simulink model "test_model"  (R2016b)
settings: Solver=VariableStepAuto  StartTime=0.0  StopTime=runtime  RelTol=1e-3
InitFcn:
  | clear mex
  | delete test_model_sfun.mexw64
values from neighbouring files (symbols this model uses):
  g = 9.81    [modelParameters.m]
  height_controlled_o = (((Rm*If +      + (((omega0_o * 2 * Rm * Kv * Kq      * Kd + 1)^2) - 1)/(4* Rm*Kv^2*Kq      * Kd))/Vb)*(Pmax- Pmin) + Pmin)    [modelParameters.m]
  If = 0.511    [modelParameters.m]
  Jreq = 4.2012e-05    [modelParameters.m]
  Jxx = 0.0130    (= 0.013)    [modelParameters.m]
  Jyy = 0.0140    (= 0.014)    [modelParameters.m]
  Jzz = 0.0285    [modelParameters.m]
  Kd = 1.0317e-7    (= 1.0317e-07)    [modelParameters.m]
  Kq = 96.3422    [modelParameters.m]
  Kt = 8.6519e-6    (= 8.6519e-06)    [modelParameters.m]
  Kv = 96.3422    [modelParameters.m]
  m = 1.244    [modelParameters.m]
  omega0_o = sqrt((m*g)/(4*Kt))    [modelParameters.m]
  omega1_o = sqrt((m*g)/(4*Kt))    [modelParameters.m]
  omega2_o = sqrt((m*g)/(4*Kt))    [modelParameters.m]
  omega3_o = sqrt((m*g)/(4*Kt))    [modelParameters.m]
  pitch_o = 0    [modelParameters.m]
  pitchrate_o = 0    [modelParameters.m]
  Pmax = 2e5    (= 200000)    [modelParameters.m]
  Pmin = 1e5    (= 100000)    [modelParameters.m]
  rhx = 0.16    [modelParameters.m]
  rhy = 0.16    [modelParameters.m]
  rhz = 0.03    [modelParameters.m]
  Rm = 0.2308    [modelParameters.m]
  roll_o = 0    [modelParameters.m]
  rollrate_o = 0    [modelParameters.m]
  Tc = 0.04    [modelParameters.m]
  Tq = 0.005    [modelParameters.m]
  Vb = 11.1    [modelParameters.m]
  x_controlled_o = 0    [modelParameters.m]
  x_o = 0    [modelParameters.m]
  x_vel_o = 0    [modelParameters.m]
  y_controlled_o = 0    [modelParameters.m]
  y_o = 0    [modelParameters.m]
  y_vel_o = 0    [modelParameters.m]
  yaw_controlled_o = 0    [modelParameters.m]
  yaw_o = 0    [modelParameters.m]
  yawrate_o = 0    [modelParameters.m]
  z_o = 0    [modelParameters.m]
  z_vel_o = 0    [modelParameters.m]
undefined symbols (not defined in the file or in its folder): DiscIntNeverNeededParam
libraries: simulink x12, vrlib x2
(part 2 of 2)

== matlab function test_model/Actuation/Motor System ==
function w_dot = motor(Vb_eff, w, Rm, Kv, Kq, Kd, If, Jreq)

% Define each motors effective battery voltage
Vb_eff_0 = Vb_eff(1);
Vb_eff_1 = Vb_eff(2);
Vb_eff_2 = Vb_eff(3);
Vb_eff_3 = Vb_eff(4);

% Determine the angular velocity of each rotor from feedback
w_0 = w(1);
w_1 = w(2);
w_2 = w(3);
w_3 = w(4);

% Determine angular acceleration of each rotor
w_0_dot = 1/(Jreq*Rm*Kq) * Vb_eff_0 - 1/(Jreq*Rm*Kq*Kv) * w_0 - 1/(Jreq*Kq)*If - (Kd/Jreq) * w_0^2;
w_1_dot = 1/(Jreq*Rm*Kq) * Vb_eff_1 - 1/(Jreq*Rm*Kq*Kv) * w_1 - 1/(Jreq*Kq)*If - (Kd/Jreq) * w_1^2;
w_2_dot = 1/(Jreq*Rm*Kq) * Vb_eff_2 - 1/(Jreq*Rm*Kq*Kv) * w_2 - 1/(Jreq*Kq)*If - (Kd/Jreq) * w_2^2;
w_3_dot = 1/(Jreq*Rm*Kq) * Vb_eff_3 - 1/(Jreq*Rm*Kq*Kv) * w_3 - 1/(Jreq*Kq)*If - (Kd/Jreq) * w_3^2;

w_dot = [w_0_dot, w_1_dot, w_2_dot, w_3_dot];

== matlab function test_model/Actuation/Rotor System







 ==
function [B_omega_dot, B_vo_dot]= rotor(w_dot, w, B_Fg, B_omega, B_vo, m, Kt, Kd, rhx, rhy, rhz, Jreq, Jxx, Jyy, Jzz)

% Create J vector
J = [Jxx,  0 ,  0 ; ...
      0 , Jyy,  0 ; ...
      0 ,  0 , Jzz;];

% Create r_hi vector
rh_0 = [-rhx; rhy; -rhz];
rh_1 = [rhx; rhy; -rhz];
rh_2 = [-rhx; -rhy; -rhz];
rh_3 = [rhx; -rhy; -rhz];

% Define vector from body frame origin to center of mass
br_oc = [0; 0; 0];

% Define 3x3 Identity Matrix
I = eye(3);

% Create gamma vectors
gamma_Ti = [0; 0; -1];
gamma_omega_03 = [0; 0; 1];  %Rotors 0 and 3 use this gamma_omega vector
gamma_omega_12 = [0; 0; -1]; %Rotors 1 and 2 use this gamma_omega vector

% Define angular velocities for each rotor
w_0 = w(1);
w_1 = w(2);
w_2 = w(3);
w_3 = w(4);

% Define angular acceleration for each rotor
w_0_dot = w_dot(1);
w_1_dot = w_dot(2);
w_2_dot = w_dot(3);
w_3_dot = w_dot(4);

% Define the rotor force in the z-direction from each rotor
B_Fr_0 = Kt * w_0 * w_0 * gamma_Ti;
B_Fr_1 = Kt * w_1 * w_1 * gamma_Ti;
B_Fr_2 = Kt * w_2 * w_2 * gamma_Ti;
B_Fr_3 = Kt * w_3 * w_3 * gamma_Ti;

% Sum up the rotor forces in the z-direction from each vector to get the
% total body force in the z-direction
B_Fr = B_Fr_0 + B_Fr_1 + B_Fr_2 + B_Fr_3;

% Define the in-plane drag and induced torque produced by each rotor
 B_Q_d0 = -1 * Kd * w_0 * w_0 * gamma_omega_03;
 B_Q_d1 = -1 * Kd * w_1 * w_1 * gamma_omega_12;
 B_Q_d2 = -1 * Kd * w_2 * w_2 * gamma_omega_12;
 B_Q_d3 = -1 * Kd * w_3 * w_3 * gamma_omega_03;

% Sum up the total in-plane drag and induced torque to get the total
% in-plane drag and induced torque on the body
B_Q_d = B_Q_d0 + B_Q_d1 + B_Q_d2 + B_Q_d3;

% Define the force lever arm torque created from the force produced by each
% rotor in the z-direction
B_Q_F0 = cross( rh_0, B_Fr_0 );
B_Q_F1 = cross( rh_1, B_Fr_1 );
B_Q_F2 = cross( rh_2, B_Fr_2 );
B_Q_F3 = cross( rh_3, B_Fr_3 );

B_Q_F = B_Q_F0 + B_Q_F1 + B_Q_F2 + B_Q_F3;

%Define the change in angular momentum torque produced by each rotor 
B_Q_L0 = -1 * Jreq * ( cross(B_omega, w_0 * gamma_omega_03) + w_0_dot * gamma_omega_03 );
B_Q_L1 = -1 * Jreq * ( cross(B_omega, w_1 * gamma_omega_12) + w_1_dot * gamma_omega_12 ); 
B_Q_L2 = -1 * Jreq * ( cross(B_omega, w_2 * gamma_omega_12) + w_2_dot * gamma_omega_12 ); 
B_Q_L3 = -1 * Jreq * ( cross(B_omega, w_3 * gamma_omega_03) + w_3_dot * gamma_omega_03 );

% Sum up the total change in angular momentum torque produced by each rotor
B_Q_L = B_Q_L0 + B_Q_L1 + B_Q_L2 + B_Q_L3;

% Define the total rotor system torque as the sum of the in-plane drag and
% induced torque, force lever arm torque, and change in angular momentum
% torques
B_Q = B_Q_d + B_Q_F + B_Q_L;

% Define the body forces in the z-direction from each vector to get the
% total body force in the z-direction
B_F = B_Fr + B_Fg; 

% Define the body frame linear velocities
B_vo_dot = (m*I)^(-1) * ( B_F - cross( B_omega, m*(B_vo + cross(B_omega, br_oc)) ) );

% Define the body frame angular velocities
B_omega_dot = J ^(-1) * ( B_Q - cross(B_omega, J * B_omega) - cross(br_oc, B_F) );

== matlab function test_model/Actuation/Aeb














 ==
function euler_rates = angular_body_earth_conversion(B_omega, euler_angles)

phi = euler_angles(1);
theta = euler_angles(2);

Aeb = [1,  sin(phi)*tan(theta), cos(phi)*tan(theta); ...
       0,      cos(phi)       ,        -sin(phi)   ; ...
       0,  sin(phi)/cos(theta), cos(phi)/cos(theta)];

   
euler_rates = Aeb * B_omega;

== matlab function test_model/Actuation/Lbe

















 ==
function [B_Fg, B_g]  = linear_earth_body_conversion(E_Fg, euler_angles, m)

phi = euler_angles(1);
theta = euler_angles(2);
psi = euler_angles(3);

Lbe = [             cos(theta)*cos(psi)              ,          cos(theta)*sin(psi)                  ,     -sin(theta)    ; ...
       sin(phi)*sin(theta)*cos(psi)-cos(phi)*sin(psi), sin(phi)*sin(theta)*sin(psi)+cos(phi)*cos(psi), sin(phi)*cos(theta); ...
       cos(phi)*sin(theta)*cos(psi)+sin(phi)*sin(psi), cos(phi)*sin(theta)*sin(psi)-sin(phi)*cos(psi), cos(phi)*cos(theta)];

B_Fg = Lbe * E_Fg;

B_g = B_Fg/m;

== matlab function test_model/     Sensors   /IMU





/






 ==
function [accelReading,gyroReading] = idealIMU(B_vo_dot, B_vo, B_Omega, B_g, r_oc, g)
%#codegen

a = B_vo_dot + cross(B_Omega,B_vo) ; % body frame acceleration 

accelReading = (a - B_g)/g ; % accelerometer reading (ideal)

gyroReading = B_Omega ; % gyroscope reading (ideal) 

end

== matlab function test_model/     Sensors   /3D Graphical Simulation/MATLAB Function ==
function y = eigenaxis_ucart(u)


if abs(u(1))< 0.0001
    u(1) = 0.0001;
end

if abs(u(2))< 0.0001
    u(2) = 0.0001;
end

if abs(u(3))< 0.0001
    u(3) = 0.0001;
end

u = [ -u(1); -u(2); u(3) ];% [Pitch, Yaw, Roll] 

C11 = cos(u(2))*cos(u(3));
C12 = cos(u(2))*sin(u(3));
C13 = -sin(u(2));
C21 = sin(u(1))*sin(u(2))*cos(u(3))-cos(u(1))*sin(u(3));
C22 = sin(u(1))*sin(u(2))*sin(u(3))+cos(u(1))*cos(u(3));
C23 = sin(u(1))*cos(u(2));
C31 = cos(u(1))*sin(u(2))*cos(u(3))+sin(u(1))*sin(u(3));
C32 = cos(u(1))*sin(u(2))*sin(u(3))-sin(u(1))*cos(u(3));
C33 = cos(u(1))*cos(u(2));
    
theta = acos(0.5*(C11+C22+C33-1));

e = [C23-C32; C31-C13; C12-C21]/(2*sin(theta));
    
y = [e; theta];

== matlab function test_model/     Sensors   /Aeb









 ==
function euler_rates_IMU = angular_body_earth_conversion(gyro_reading, euler_angles_filtered)

phi = euler_angles_filtered(1);
theta = euler_angles_filtered(2);

Aeb = [1, sin(phi)*tan(theta), cos(phi)*tan(theta); ...
       0,     cos(phi)       ,        -sin(phi)   ; ...
       0,  sin(phi)/cos(theta), cos(phi)/cos(theta)];

   
euler_rates_IMU = Aeb * gyro_reading;

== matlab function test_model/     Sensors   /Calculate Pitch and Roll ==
function [accel_pitch, accel_roll] = getPitchAndRoll(accel_reading, accel_roll_prev)

mag = norm(accel_reading);

% x_accel = accel_reading(1)/mag;
% y_accel = accel_reading(2)/mag;
% z_accel = accel_reading(3)/mag;

x_accel = accel_reading(1);
y_accel = accel_reading(2);
z_accel = accel_reading(3);

accel_pitch = atan(x_accel/sqrt(y_accel^2 + z_accel^2));

accel_roll = atan2( -y_accel,(sign(-z_accel)*sqrt(z_accel^2 + (1/100)*x_accel^2)) );
unwrapped_roll = unwrap([accel_roll_prev accel_roll]);
accel_roll = unwrapped_roll(2);

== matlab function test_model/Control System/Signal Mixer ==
function P  = signal_mixer(height_controlled, y_controlled, x_controlled, yaw_controlled)

controller_outputs = [ height_controlled; x_controlled; y_controlled; yaw_controlled ];
signal_mixer = [ 1, -1, -1, -1; ... 
                 1,  1, -1,  1; ...
                 1, -1,  1,  1; ...
                 1,  1,  1, -1 ];

% signal_mixer = [ 1,  1, -1, -1; ... 
%                  1, -1, -1,  1; ...
%                  1,  1,  1,  1; ...
%                  1, -1,  1, -1 ];
             
P = signal_mixer * controller_outputs;

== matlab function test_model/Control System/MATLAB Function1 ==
function [z_corr, y_cor, x_corr, yaw_corr, pid_y_out, pid_roll_out] = c_controller(set_x, set_y, set_z, set_yaw, ...
    cur_x, cur_y, cur_z, ...
    cur_phi, cur_theta, cur_psi, ...
    cur_phi_d, cur_theta_d, cur_psi_d, vrpn_id, Tc)

out_z = -1;
out_y = -1;
out_x = -1;
out_yaw = -1;
c_pid_y = -1;
c_pid_roll = -1;

coder.ceval('c_controller', vrpn_id, Tc, set_x, set_y, set_z, set_yaw, ...
                    cur_x, cur_y, cur_z, ...
                    cur_phi, cur_theta, cur_psi, ...
                    cur_phi_d, cur_theta_d, cur_psi_d, ...
                    coder.wref(out_z), coder.wref(out_y), coder.wref(out_x), coder.wref(out_yaw), ...
                    coder.wref(c_pid_y), coder.wref(c_pid_roll));

z_corr = out_z;
y_cor = out_y;
x_corr = out_x;
pid_y_out = c_pid_y;
pid_roll_out = c_pid_roll;
yaw_corr = out_yaw;

== matlab function test_model/     Sensors   /Aeb









1 ==
function euler_rates_IMU = angular_body_earth_conversion(gyro_reading, euler_angles_filtered)

phi = euler_angles_filtered(1);
theta = euler_angles_filtered(2);
psi = NaN;

phi_dot = -1;
theta_dot = -1;
psi_dot = -1;

p = gyro_reading(1);
q = gyro_reading(2);
r = gyro_reading(3);

coder.ceval( 'aeb_mat', p, q, r, phi, theta, psi, coder.wref(phi_dot), ...
    coder.wref(theta_dot), coder.wref(psi_dot) );

   
euler_rates_IMU = [phi_dot; theta_dot; psi_dot];

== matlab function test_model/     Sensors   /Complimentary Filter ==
%function euler_angles_IMU  = complimentaryFilter(accel_pitch, accel_roll, euler_angles_gyro, prev_euler_angles_IMU)
function euler_angles_IMU  = complimentaryFilter(accel_pitch, accel_roll, euler_rates_gyro, prev_euler_angles)

% LOOP_TIME = 5*10^-3;
% 
% prev_phi = prev_euler_angles_IMU(1);
% prev_theta = prev_euler_angles_IMU(2);
% 
% phi_dot_gyro = euler_angles_gyro(1);
% theta_dot_gyro = euler_angles_gyro(2);

% phi = 0.98 * ( prev_phi + phi_dot_gyro * LOOP_TIME ) + 0.02 * accel_roll;
% theta = 0.98 * ( prev_theta + theta_dot_gyro * LOOP_TIME) + 0.02 * accel_pitch;
k_gyro = 0.98; 
k_accel = 1-k_gyro; 

Ts = 0.005; % 5 milliseconds

prev_phi = prev_euler_angles(1);
prev_theta = prev_euler_angles(2);

prev_phi_dot = euler_rates_gyro(1);
prev_theta_dot = euler_rates_gyro(2);

integrated_phi_gyro = Ts * prev_phi_dot + prev_phi;
integrated_theta_gyro = Ts * prev_theta_dot + prev_theta;

phi = k_gyro * integrated_phi_gyro + k_accel * accel_roll;
theta = k_gyro * integrated_theta_gyro + k_accel * accel_pitch;

euler_angles_IMU = [phi; theta];
